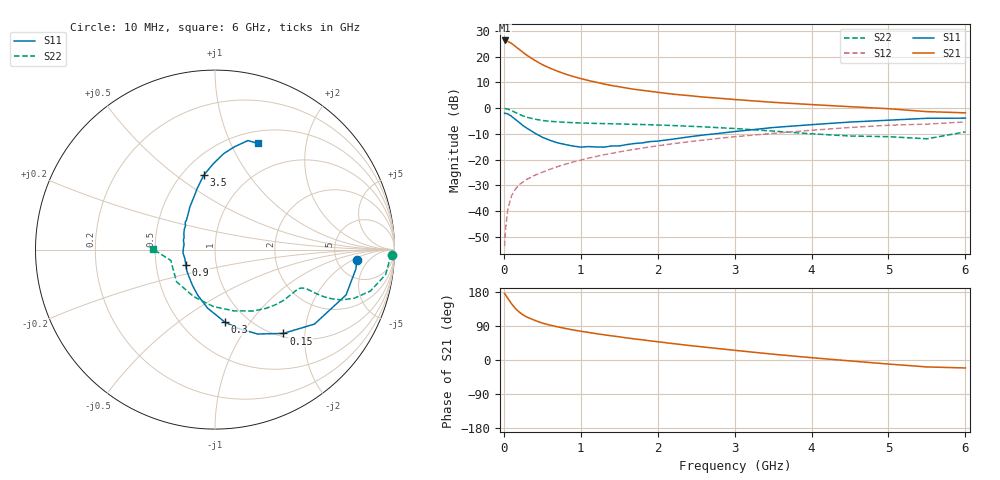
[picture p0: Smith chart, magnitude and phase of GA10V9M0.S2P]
! Infineon Technologies  Discrete & RF Semiconductors
! BF775
! Si NPN RF Bipolar Junction Transistor in SOT23
! VCE = 10 V  IC = 9 mA
! Common Emitter S-Parameters:  May  1996
# GHz  S  MA  R  50
!  f  S11  S21  S12  S22
! GHz  MAG  ANG  MAG  ANG  MAG  ANG  MAG  ANG
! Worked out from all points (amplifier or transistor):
!   36 points, 10 MHz to 6 GHz, reference 50 ohm
!   highest |S21| = 26.2 dB at 10 MHz (marker M1)
!   |S21| within 3 dB of that: start of sweep to 180.1 MHz
!   unconditionally stable (mu >= 1): 679.4 MHz to 2.802 GHz
!   at 250 MHz: K = 0.63, MSG = 25.1 dB, |S12| = -28.7 dB
!   at 1.4 GHz: K = 1.09, MAG = 11.3 dB, |S12| = -17.6 dB
!   at 6 GHz: K = 0.88, MSG = 1.8 dB, |S12| = -5.3 dB
!   S11 on the Smith chart (normalised r, x): 10 MHz: 7.91, -2.35; 150 MHz: 1.06, -1.55; 300 MHz: 0.79, -0.76; 900 MHz: 0.71, -0.12; 3.5 GHz: 0.63, +0.64; 6 GHz: 0.64, +1.28
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0.01  0.7921 -4.0  20.5 175.9  0.0021 93.5  0.9879 -1.6
0.02  0.7925 -7.8  20.1 172.5  0.0041 85.9  0.9751 -3.4
0.05  0.7726 -19.1  19.63 163.1  0.0106 80.5  0.9608 -8.3
0.1  0.6925 -36.8  18.01 148.5  0.02 73.6  0.8966 -14.9
0.15  0.6024 -50.8  15.68 136.0  0.0268 67.6  0.8225 -19.2
0.2  0.527 -63.2  13.78 126.5  0.0327 64.5  0.7585 -21.7
0.25  0.456 -73.8  12.03 118.9  0.0369 62.7  0.7036 -22.9
0.3  0.4076 -82.3  10.56 113.3  0.0416 62.7  0.6635 -23.4
0.4  0.3288 -97.2  8.462 104.8  0.0496 62.4  0.611 -23.5
0.5  0.2721 -110.6  6.964 97.4  0.0571 63.6  0.5757 -23.3
0.6  0.2369 -121.7  5.951 92.1  0.0652 63.7  0.5546 -23.2
0.7  0.2117 -132.5  5.179 87.4  0.0734 64.9  0.5408 -23.5
0.9  0.1833 -152.8  4.104 79.3  0.0902 65.0  0.5213 -24.4
1.1  0.1793 -173.9  3.431 72.8  0.107 65.1  0.5091 -26.2
1.3  0.1749 170.4  2.936 66.6  0.1243 64.3  0.5003 -28.2
1.6  0.1962 152.1  2.438 58.2  0.1502 62.9  0.4873 -32.0
2.2  0.2502 126.6  1.862 43.3  0.204 58.8  0.4591 -41.5
2.8  0.3238 110.5  1.551 29.9  0.2593 53.4  0.4164 -53.5
3.5  0.4198 98.6  1.294 15.3  0.3241 45.8  0.3581 -72.6
4.5  0.5363 84.9  1.065 -2.4  0.4203 33.9  0.2874 -114.6
5.5  0.6344 73.2  0.854 -18.3  0.4891 18.8  0.2537 -166.2
6  0.6381 67.9  0.809 -21.0  0.5402 14.7  0.3457 179.5
